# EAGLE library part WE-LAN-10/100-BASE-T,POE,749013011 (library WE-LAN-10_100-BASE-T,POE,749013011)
LAN-Transformer WE-LAN 10/100 Base Tx - Compliant with IEEE 802.3 standards - SMD -- Ethernet -- Power over Ethernet -- 1 Gigabit Ethernet -- Compliant with most IC's for ethernet applications like Intel, AMD, Globespan and Realtek -- Hub, Router, Switch
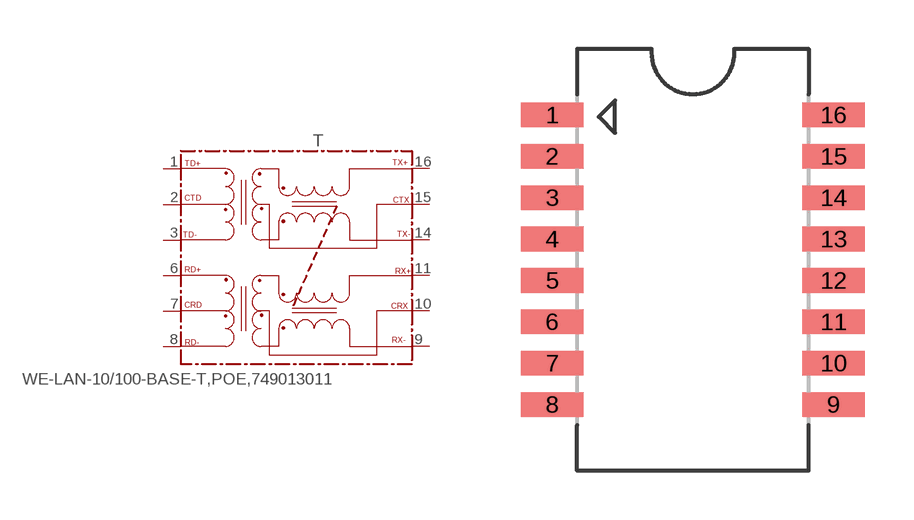
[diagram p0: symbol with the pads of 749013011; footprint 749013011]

Designator prefix T

## WE-LAN-10/100-BASE-T,POE,749013011 (MPN: 749013011; OC_FARNELL: 1636349; OC_NEWARK: 08P2943; PACKAGE: 10/100/Base-T PoE; SUPPLIER: Wuerth Elektronik)  [749013011]
1  TD+
2  CTD
3  TD-
6  RD+
7  CRD
8  RD-
9  RX-
10  CRX
11  RX+
14  TX-
15  CTX
16  TX+

## Footprint 749013011 (pad centres in mm)
MAX Height = 5.33mm
smd 1.91 x 0.76: 1 -4.317,4.445; 2 -4.317,3.175; 3 -4.317,1.905; 4 -4.317,0.635; 5 -4.317,-0.635; 6 -4.317,-1.905; 7 -4.317,-3.175; 8 -4.317,-4.445; 9 4.317,-4.445; 10 4.317,-3.175; 11 4.317,-1.905; 12 4.317,-0.635; 13 4.317,0.635; 14 4.317,1.905; 15 4.317,3.175; 16 4.317,4.445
